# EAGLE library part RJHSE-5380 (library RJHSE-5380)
Jack Modular Connector 8p8c (RJ45, Ethernet) 90 Angle (Right) Shielded, EMI Finger , 125VAC , 1.5A , -55C ~ 85C Source: Datasheet
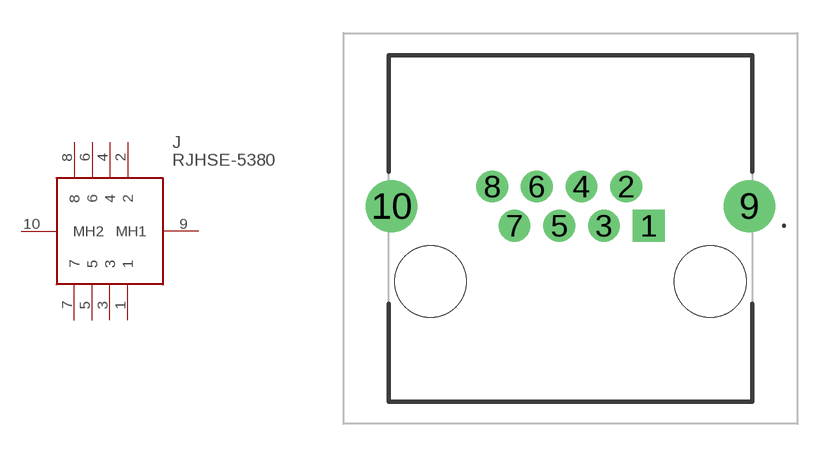
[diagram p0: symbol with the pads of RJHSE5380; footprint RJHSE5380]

Designator prefix J

## RJHSE-5380 (Description: Jack Modular Connector 8p8c (RJ45, Ethernet) 90 Angle (Right) Shielded, EMI Finger , 125VAC , 1.5A , -55C ~ 85C; Height: 13.716mm; Manufacturer_Name: Amphenol Communications Solutions; Manufacturer_Part_Number: RJHSE-5380)  [RJHSE5380]
1  1
2  2
3  3
4  4
5  5
6  6
7  7
8  8
9  MH1
10  MH2

## Footprint RJHSE5380 (pad centres in mm)
RJHSE-5380-2
drill 0.89 pad 1.446 square: 1 0,0
drill 0.89 pad 1.446: 2 -1.02,1.78; 3 -2.03,0; 4 -3.05,1.78; 5 -4.06,0; 6 -5.08,1.78; 7 -6.09,0; 8 -7.11,1.78
drill 1.57 pad 2.355: 9 4.58,0.89; 10 -11.68,0.89
hole 3.25 at 2.8,-2.54
hole 3.25 at -9.9,-2.54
